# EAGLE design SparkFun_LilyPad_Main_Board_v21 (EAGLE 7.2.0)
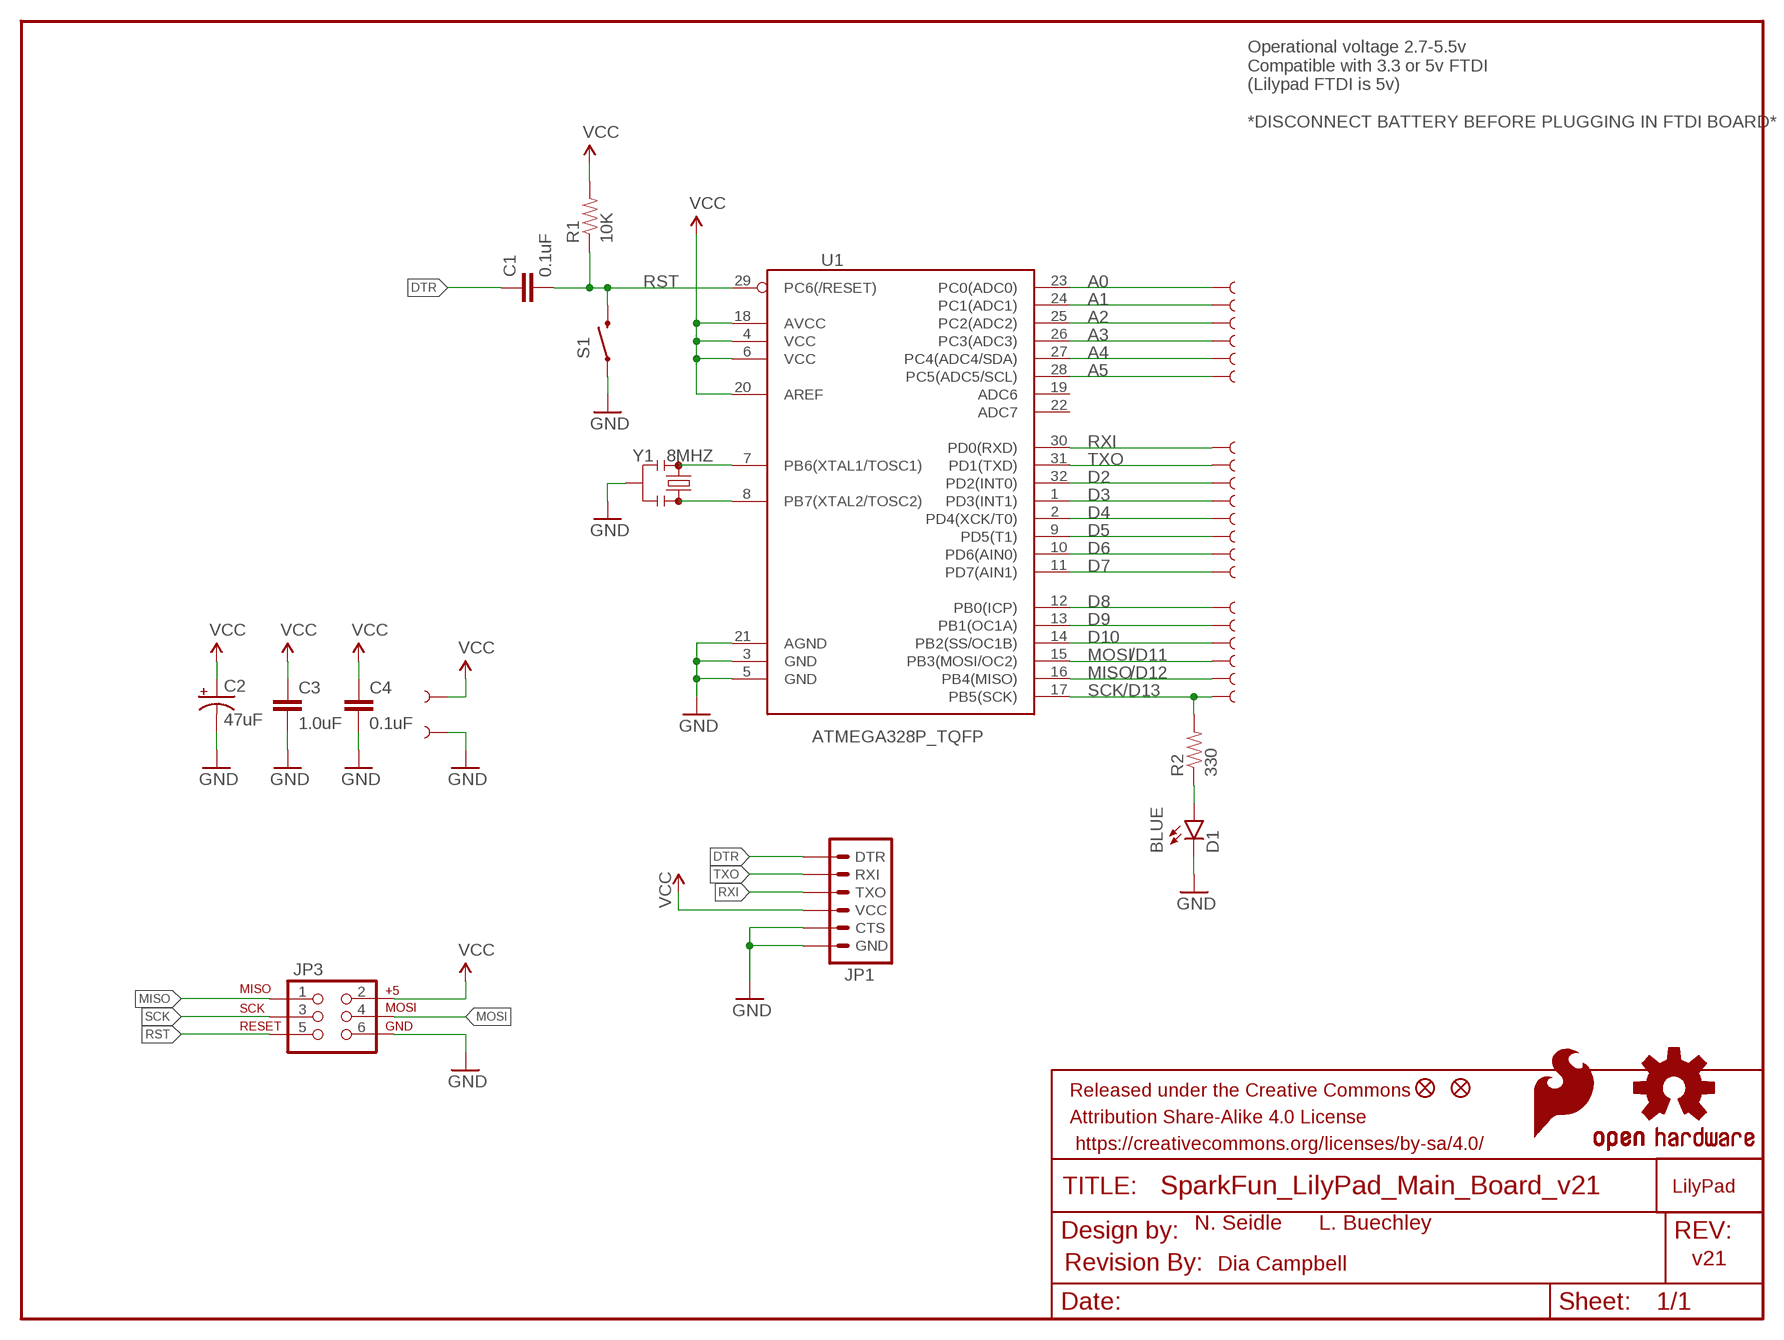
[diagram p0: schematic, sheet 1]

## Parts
$0000003  LOGO-LPLPA  [LOGO-LPA]
C1  0.1uF  0.1UF-25V(+80/-20%)(0603)  [0603-CAP]
C2  47uF  47UF-10V-10%(TANT)  [EIA3528]
C3  1.0uF  1.0UF-16V-10%(0603)  [0603-CAP]
C4  0.1uF  0.1UF-25V(+80/-20%)(0603)  [0603-CAP]
D1  BLUE  LED-BLUE0603  [LED-0603]
FID1  FIDUCIALUFIDUCIAL  [MICRO-FIDUCIAL]
FID2  FIDUCIALUFIDUCIAL  [MICRO-FIDUCIAL]
FRAME1  FRAME-LETTER  [CREATIVE_COMMONS]
GND  SEWTAP9  [PETAL-LONG-1-2SIDE]
JP1  ARDUINO_SERIAL_PROGRAMSMD  [1X06-SMD]
JP3  FEMALE 2x3  AVR_SPI_PRG_6NS  [2X3-NS]
LOGO1  SFE_LOGO_FLAME.3COP  [SFE_LOGO_FLAME_COPPER_.3]
LOGO2  OSHW-LOGO-COPPERM  [OSHW-LOGO-M]
R1  10K  10KOHM-1/10W-1%(0603)0603  [0603-RES]
R2  330  330OHM1/10W1%(0603)  [0603-RES]
S1  SWITCH-MOMENTARY-2SMD-REDUNDANT  [TACTILE-SWITCH-SMD]
U1  ATMEGA328P_TQFP  [TQFP32-08]
U$1  SEWTAP9  [PETAL-LONG-1-2SIDE]
U$2  SEWTAP9  [PETAL-LONG-1-2SIDE]
U$3  SEWTAP9  [PETAL-LONG-1-2SIDE]
U$4  SEWTAP9  [PETAL-LONG-1-2SIDE]
U$5  SEWTAP9  [PETAL-LONG-1-2SIDE]
U$6  SEWTAP9  [PETAL-LONG-1-2SIDE]
U$7  SEWTAP9  [PETAL-LONG-1-2SIDE]
U$8  SEWTAP9  [PETAL-LONG-1-2SIDE]
U$9  SEWTAP9  [PETAL-LONG-1-2SIDE]
U$10  SEWTAP9  [PETAL-LONG-1-2SIDE]
U$11  SEWTAP9  [PETAL-LONG-1-2SIDE]
U$12  SEWTAP9  [PETAL-LONG-1-2SIDE]
U$13  SEWTAP9  [PETAL-LONG-1-2SIDE]
U$14  SEWTAP9  [PETAL-LONG-1-2SIDE]
U$15  SEWTAP9  [PETAL-LONG-1-2SIDE]
U$16  SEWTAP9  [PETAL-LONG-1-2SIDE]
U$17  SEWTAP9  [PETAL-LONG-1-2SIDE]
U$18  SEWTAP9  [PETAL-LONG-1-2SIDE]
U$19  SEWTAP9  [PETAL-LONG-1-2SIDE]
U$20  SEWTAP9  [PETAL-LONG-1-2SIDE]
U$21  SEWTAP9  [PETAL-LONG-1-2SIDE]
U$22  REVISION  [REVISION]
Y1  8MHZ  RESONATOR8MHZ  [RESONATOR-SMD]

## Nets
A0: U1.23(PC0(ADC0)) U$1.1
A1: U1.24(PC1(ADC1)) U$2.1
A2: U1.25(PC2(ADC2)) U$3.1
A3: U1.26(PC3(ADC3)) U$4.1
A4: U1.27(PC4(ADC4/SDA)) U$5.1
A5: U1.28(PC5(ADC5/SCL)) U$6.1
D2: U1.32(PD2(INT0)) U$9.1
D3: U1.1(PD3(INT1)) U$10.1
D4: U1.2(PD4(XCK/T0)) U$11.1
D5: U1.9(PD5(T1)) U$12.1
D6: U1.10(PD6(AIN0)) U$13.1
D7: U1.11(PD7(AIN1)) U$14.1
D8: U1.12(PB0(ICP)) U$15.1
D9: U1.13(PB1(OC1A)) U$16.1
D10: U1.14(PB2(SS/OC1B)) U$17.1
DTR: C1.1 JP1.1(DTR)
GND [VCC]: C2.C(-) C3.2 C4.2 D1.C GND.1 JP1.5(CTS) JP1.6(GND) JP3.6 S1.1 S1.2 U1.3(GND) U1.5(GND) U1.21(AGND) Y1.2
MISO: JP3.1 U1.16(PB4(MISO)) U$19.1
MOSI: JP3.4 U1.15(PB3(MOSI/OC2)) U$18.1
N$1: U1.7(PB6(XTAL1/TOSC1)) Y1.1
N$2: D1.A R2.1
N$3: U1.8(PB7(XTAL2/TOSC2)) Y1.3
RST: C1.2 JP3.5 R1.1 S1.3 S1.4 U1.29(PC6(/RESET))
RXI: JP1.3(TXO) U1.30(PD0(RXD)) U$7.1
SCK: JP3.3 R2.2 U1.17(PB5(SCK)) U$21.1
TXO: JP1.2(RXI) U1.31(PD1(TXD)) U$8.1
VCC [VCC]: C2.A(+) C3.1 C4.1 JP1.4(VCC) JP3.2 R1.2 U1.4(VCC) U1.6(VCC) U1.18(AVCC) U1.20(AREF) U$20.1
Unconnected: U1.19(ADC6) U1.22(ADC7)

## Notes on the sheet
- Operational voltage 2.7-5.5v
  Compatible with 3.3 or 5v FTDI
  (Lilypad FTDI is 5v)
  
  *DISCONNECT BATTERY BEFORE PLUGGING IN FTDI BOARD*
- /D11
- /D12
- /D13
- N. Seidle | L. Buechley
- Dia Campbell | v21

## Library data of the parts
$0000003 = LilyPad-Wearables:LOGO-LP
C1 C4 = SparkFun-Capacitors:0.1UF-25V(+80/-20%)(0603): CAP-00810; PROD_ID: CAP-00810
C2 = SparkFun-Capacitors:47UF-10V-10%(TANT): CAP-08310; PROD_ID: CAP-08310
C3 = SparkFun-Capacitors:1.0UF-16V-10%(0603): CAP-00868; PROD_ID: CAP-00868
D1 = SparkFun-LED:LED-BLUE: Blue LEDs for production use; PROD_ID: DIO-08575
FID1 FID2 = SparkFun-Aesthetics:FIDUCIAL: Fiducial Alignment Points
FRAME1 = SparkFun-Aesthetics:FRAME-LETTER: Schematic Frame; DESIGNER: NAME; VERSION: v01
GND U$1-U$21 = LilyPad-Wearables:SEWTAP: Sew Taps for LilyPad Boards.
JP1 = SparkFun-Connectors:ARDUINO_SERIAL_PROGRAM: FTDI connector footprints; PROD_ID: CONN-08971
JP3 = SparkFun-Connectors:AVR_SPI_PRG_6: AVR ISP 6 Pin This is the reduced ISP connector for AVR programming. Common on Arduino. This footprint will take up less PCB space and can be used with a 10-pin to 6-pin adapter such as SKU: BOB-08508 **Special note about "TEST_POINT" package. The stop mask is on the top side, so if you want your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
LOGO1 = SparkFun-Aesthetics:SFE_LOGO_FLAME: SFE Logo, flame only
LOGO2 = SparkFun-Aesthetics:OSHW-LOGO-COPPER: Open Source Hardware Logo
R1 = SparkFun-Resistors:10KOHM-1/10W-1%(0603): RES-00824; PROD_ID: RES-00824
R2 = SparkFun-Resistors:330OHM1/10W1%(0603): RES-00818; PROD_ID: RES-00818
S1 = SparkFun-Electromechanical:SWITCH-MOMENTARY-2: Various NO switches- pushbuttons, reed, etc; PROD_ID: SWCH-08247
U1 = SparkFun-DigitalIC:ATMEGA328P_TQFP; PROD_ID: IC-09069
U$22 = SparkFun-Aesthetics:REVISION
Y1 = SparkFun-FreqCtrl:RESONATOR: Resonator Small SMD resonator. Used, eg, on the Arduino Pro/ Pro Mini boards. 8MHz- XTAL-08895 16MHz- XTAL-08900; PROD_ID: XTAL-08895

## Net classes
0 Default: width 0.203 mm
1 VCC: width 0.305 mm

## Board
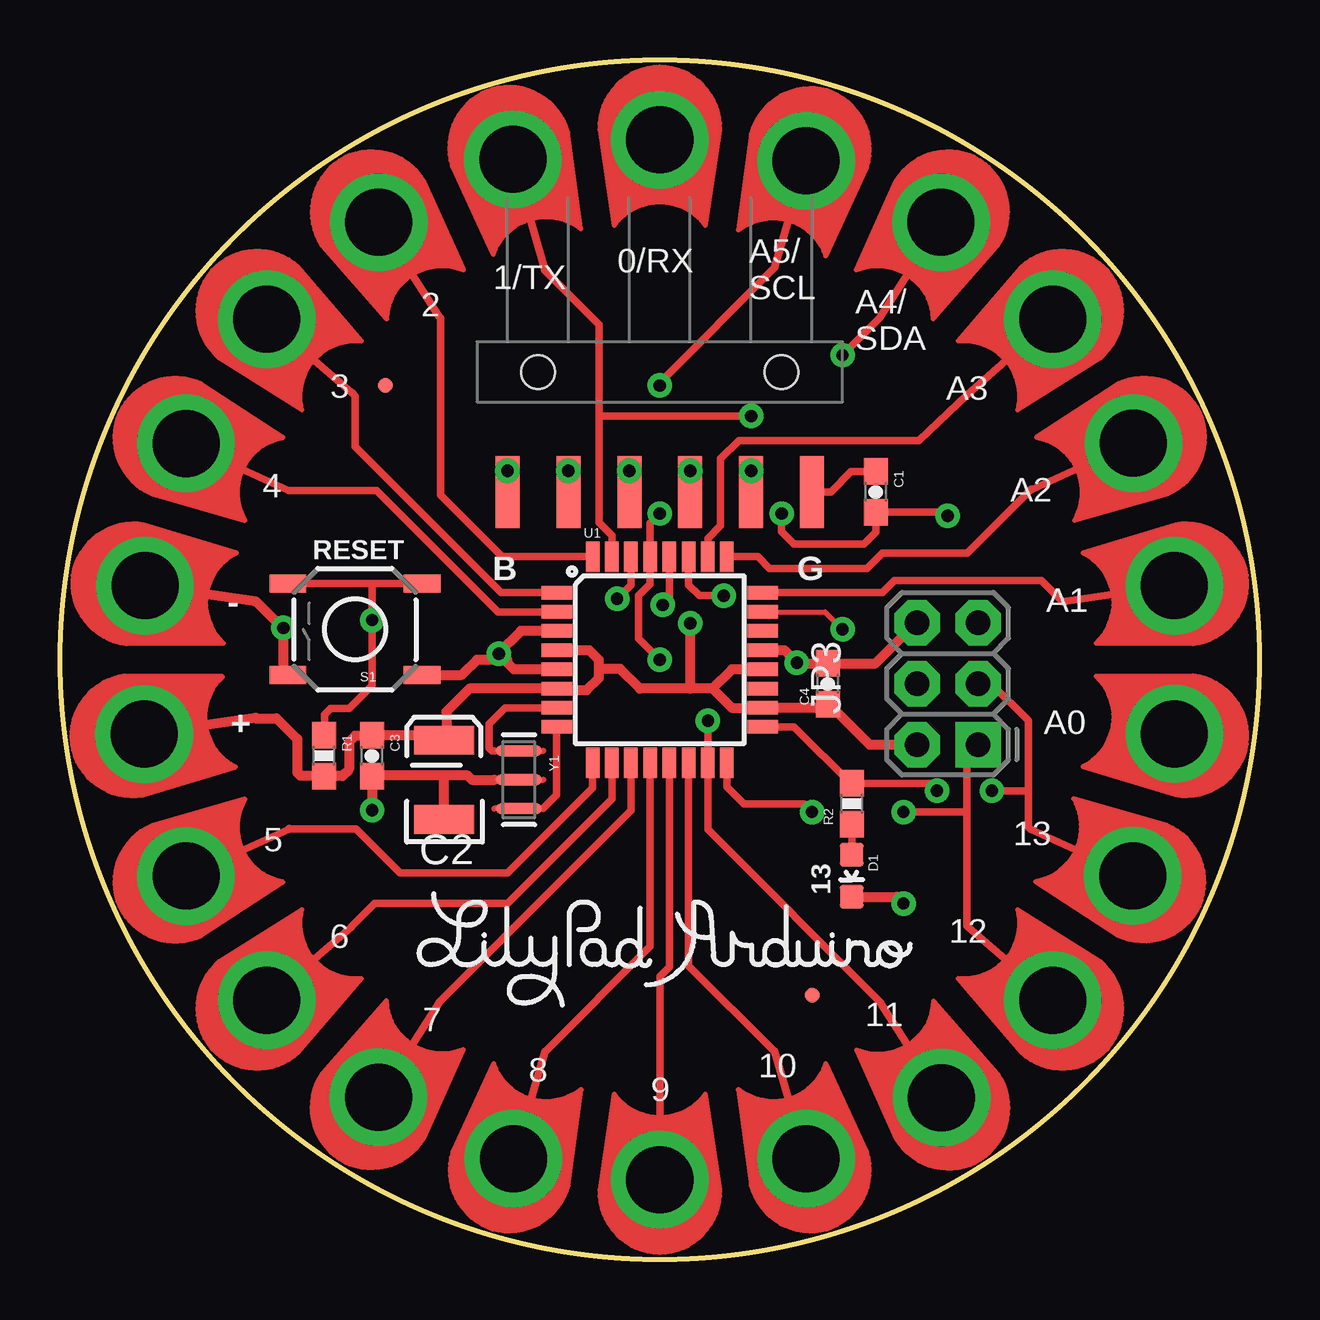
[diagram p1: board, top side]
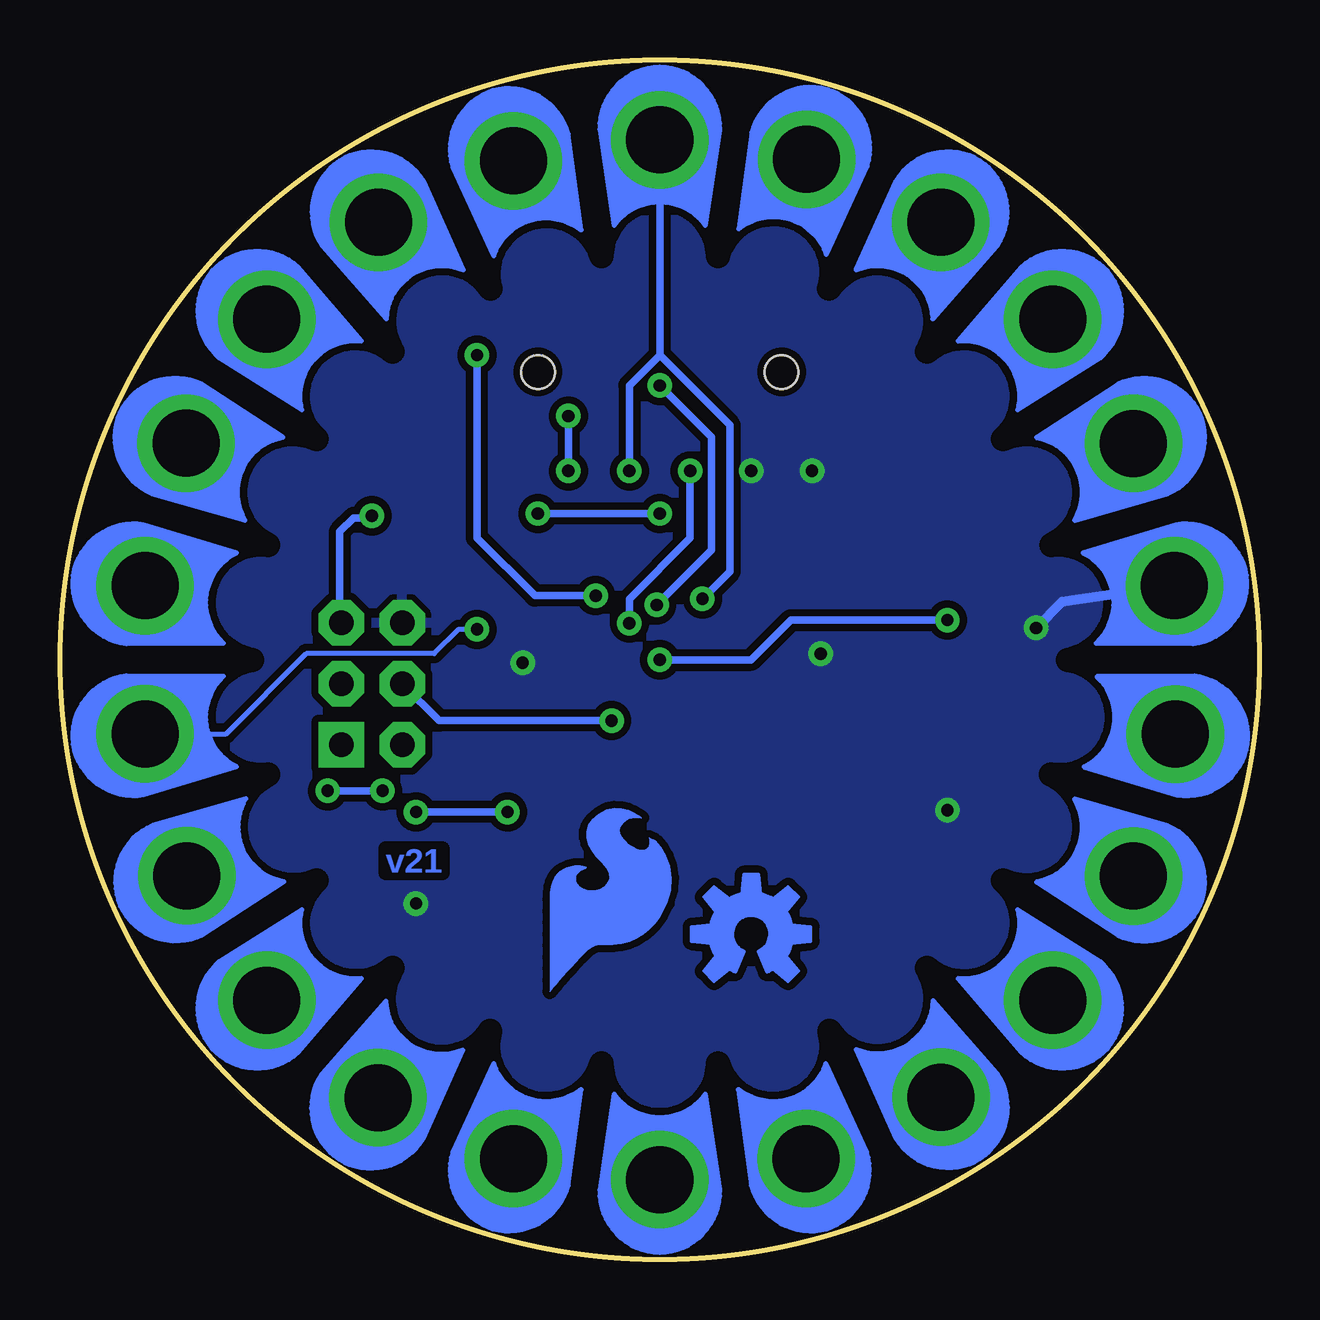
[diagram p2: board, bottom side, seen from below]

Size 50 x 50 mm. Coordinates in mm from the lower left corner, seen from the top.
Outline: circle at 25,25 radius 25
Copper layers (1*16): Top 0.035mm / dielectric 1.5mm / Bottom 0.035mm
Design rules "SparkFun-2-layer": minimum track width 7mil, minimum drill 15mil, track to track 8mil, track to pad 8mil, pad to pad 8mil, via to via 8mil, smd to smd 8mil, copper to edge 8mil, drill to drill 8mil, minimum pad ring 12mil, minimum via ring 10mil, stop-mask expansion 4mil, vias tented up to drill 20mil, thermal gap 10mil
bRestrict: area 2.4,2.4 to 47.6,47.6; area 21,42.8 to 23.5,44; area 31.6,41.3 to 34.4,43; area 36.3,38.4 to 38.9,40.7; area 40,34.1 to 42,36.9; area 42.2,29.2 to 43.6,31.8; area 42.8,23.9 to 44,26.2; area 42.2,18.2 to 43.7,20.9; area 36.3,9.4 to 39,11.7; area 31.7,7 to 34.5,8.7; area 26.5,6 to 28.9,7.3; area 21.1,6 to 23.6,7.3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; 22 lines

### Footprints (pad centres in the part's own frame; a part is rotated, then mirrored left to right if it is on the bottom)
0603-CAP = smd 1.1 x 1: 1 -0.85,0; 2 0.85,0
EIA3528 = smd 1.2 x 2.5: A 1.65,0; C -1.65,0
LED-0603 = smd 1 x 1: A 0,-0.877; C 0,0.877
MICRO-FIDUCIAL = smd 0.635 x 0.635: 1 0,0
PETAL-LONG-1-2SIDE = drill 2.794 pad 4.064: 1 0.03,0
1X06-SMD = smd 1 x 3: 1 -6.35,5; 2 -3.81,5; 3 -1.27,5; 4 1.27,5; 5 3.81,5; 6 6.35,5 | hole 1.4: -5.08,0; 5.08,0
2X3-NS = drill 1.016 pad 1.88 square: 1 -2.54,-1.27 | drill 1.016 pad 1.88 octagon: 2 -2.54,1.27; 3 0,-1.27; 4 0,1.27; 5 2.54,-1.27; 6 2.54,1.27
0603-RES = smd 1.1 x 1: 1 -0.85,0; 2 0.85,0
TACTILE-SWITCH-SMD = smd 1.524 x 0.762: 1 -2.794,1.905; 2 2.794,1.905; 3 -2.794,-1.905; 4 2.794,-1.905
TQFP32-08 = smd 1.27 x 0.559: 1 -4.293,2.8; 2 -4.293,2; 3 -4.293,1.2; 4 -4.293,0.4; 5 -4.293,-0.4; 6 -4.293,-1.2; 7 -4.293,-2; 8 -4.293,-2.8; 17 4.293,-2.8; 18 4.293,-2; 19 4.293,-1.2; 20 4.293,-0.4; 21 4.293,0.4; 22 4.293,1.2; 23 4.293,2; 24 4.293,2.8 | smd 0.559 x 1.27: 9 -2.8,-4.293; 10 -2,-4.293; 11 -1.2,-4.293; 12 -0.4,-4.293; 13 0.4,-4.293; 14 1.2,-4.293; 15 2,-4.293; 16 2.8,-4.293; 25 2.8,4.293; 26 2,4.293; 27 1.2,4.293; 28 0.4,4.293; 29 -0.4,4.293; 30 -1.2,4.293; 31 -2,4.293; 32 -2.8,4.293
RESONATOR-SMD = smd 0.45 x 1.905: 1 -1.2,0; 2 0,0; 3 1.2,0

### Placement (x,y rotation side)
$0000003  25,13.3 0 top
C1  34,32 270 top
C2  16,20 90 top
C3  13,21 270 top
C4  32,24 90 top
D1  33,16 180 top
FID1  13.57,36.43 0 top
FID2  31.35,11.03 0 top
FRAME1  not placed on the board
GND  3.52,28.09 351.8 top
JP1  25,37 180 top
JP3  37,24 90 top
LOGO1  30.08,11.03 0 bottom
LOGO2  21.19,13.57 0 bottom
R1  11,21 270 top
R2  33,19 90 top
S1  12.3,26.27 180 top
U1  25,25 0 top
U$1  46.48,21.91 171.8 top
U$2  46.48,28.09 188.2 top
U$3  44.77,34.04 204.5 top
U$4  41.4,39.21 220.9 top
U$5  36.74,43.26 237.3 top
U$6  31.11,45.83 253.7 top
U$7  25,46.7 270 top
U$8  18.87,45.89 286.3 top
U$9  13.27,43.26 302.7 top
U$10  8.6,39.21 319.1 top
U$11  5.23,34.03 335.5 top
U$12  5.23,15.97 24.5 top
U$13  8.6,10.79 40.9 top
U$14  13.26,6.74 57.3 top
U$15  18.89,4.17 73.7 top
U$16  25,3.3 90 top
U$17  31.11,4.17 106.3 top
U$18  36.76,6.72 122.7 top
U$19  41.4,10.79 139.1 top
U$20  3.48,21.9 8.2 top
U$21  44.74,15.98 155.5 top
U$22  not placed on the board
Y1  19.13,20 270 top

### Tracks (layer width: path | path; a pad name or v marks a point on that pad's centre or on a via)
A0  (via drill 0.51)
  Top 0.203: U1.23 31.89,27 v32.62,26.27
  Bottom 0.203: v32.62,26.27 33.38,26.27 34.4,25.25 39.73,25.25 43.07,21.91 U$1.1
A1
  Top 0.305: U$2.1 41.83,27.42 41.82,27.42 41.8,27.4 40.9,28.3 34.78,28.3 34.28,27.8 U1.24
A2
  Top 0.305: U$3.1 40.5,32.1 40.5,32.11 40.49,32.11 37.83,29.45 34.27,29.45 33.64,28.81 29.57,28.81 29.09,29.29 U1.25
A3
  Top 0.305: U1.26 27,30.05 27.54,30.59 27.54,33.38 28.3,34.14 35.8,34.14 37.83,36.05 U$4.1
A4  (via drill 0.51)
  Top 0.305: U$5.1 34.2,39.3 34.2,39.28 v32.62,37.7 | U1.27 26.2,28.12 26.65,27.67 v27.67,27.67
  Bottom 0.305: v27.67,27.67 30.21,27.67 32.62,30.08 v32.62,37.7
A5  (via drill 0.51)
  Top 0.305: U$6.1 29.8,41.4 29.8,41.36 25,36.56 v25,36.43 | U1.28 25.4,27.56 v25.13,27.29
  Bottom 0.305: v25,36.43 22.84,34.27 22.84,29.57 v25.13,27.29
D2
  Top 0.305: U$9.1 15.8,39.3 15.86,39.24 15.86,31.86 18.42,29.29 U1.32
D3
  Top 0.305: U$10.1 12.16,36.13 12.17,36.13 12.3,36 12.3,33.89 18.39,27.8 U1.1
D4
  Top 0.305: U$11.1 9.54,32.06 9.56,32.06 13.19,32.06 18.25,27 U1.2
D5
  Top 0.305: U$12.1 9.54,17.93 9.54,17.95 9.56,17.96 9.58,17.94 12.35,17.94 14.18,16.11 18.65,16.11 22.2,19.66 U1.9
D6
  Top 0.305: U$13.1 12.15,13.87 12.15,13.88 13.11,14.84 18.65,14.84 23,19.19 U1.10
D7
  Top 0.305: U$14.1 15.8,10.7 15.8,10.72 23.8,18.72 U1.11
D8
  Top 0.305: U$15.1 20.21,8.68 20.24,8.68 24.6,13.04 U1.12
D9
  Top 0.305: 25,11.79 U$16.1 | 25,11.79 25,8 | U1.13 25.4,12.19 25,11.79
D10
  Top 0.305: U$17.1 29.79,8.69 29.75,8.69 26.2,12.24 U1.14
DTR
  Top 0.305: JP1.1 32.13,32 32.98,32.85 C1.1
GND  (via drill 0.51)
  Top 0.305: C4.2 32,24.8 | v13,18.74 v13.01,18.73 | C2.C 16,18.41 16.03,18.45 15.98,18.5 | v18.29,25.25 18.32,25.28 | 13.06,20.17 13.04,20.15 C3.2 | 18.27,25.25 v18.29,25.25 | JP1.6 v18.65,32.87 | JP1.5 v21.19,32.87 | 9.3,26.3 9.31,26.31 v9.31,26.33 9.27,26.33 | 8.18,27.42 8.17,27.42 | 9.3,24.57 S1.2 | v18.29,25.25 18.4,25.25 18.65,25
  Top 0.406: 8.17,27.42 GND.1 | C3.2 v13,18.74 | 15.98,20.17 17,20.17 17.17,20 18.11,20 | 15.98,20.17 15.98,18.5 | 15.98,20.17 13.06,20.17 | 9.27,26.33 8.18,27.42 | U1.5 18.92,24.6 18.27,25.25 19.21,26.2 U1.3 | U1.21 30.19,25.4 v30.71,24.87 30.74,24.85 C4.2 33.99,24.85 35.67,26.52 | 9.3,26.3 9.3,24.57 | 18.65,25 17.38,25 16.74,24.36 S1.1 | D1.C 34.88,15.12 v35.16,14.84
  Bottom 0.406: GND.1 8.24,27.41 v9.31,26.33
  pour Bottom (isolate 0.305): -1,51 51,51 51,-1 -1,-1
MISO  (via drill 0.51)
  Top 0.305: U$19.1 37.85,13.87 37.82,13.9 37.8,13.9 37.8,18.65 | JP3.1 37.8,20.99 37.8,18.65 | U1.16 27.8,19.7 28.5,19 31,19 v31.35,18.65 | v35.16,18.65 37.8,18.65
  Bottom 0.305: v31.35,18.65 v35.16,18.65
MOSI  (via drill 0.51)
  Top 0.305: U$18.1 34.2,10.7 34.2,10.72 27,17.92 U1.15 v27,22.45 v27.01,22.46
  Bottom 0.305: JP3.4 35.74,24.01 | JP3.4 | v27.01,22.46 34.2,22.46 JP3.4
N$1
  Top 0.305: U1.7 18.55,23 17.89,22.33 17.89,21.32 18,21.2 18.11,21.2
N$2
  Top 0.305: 33,16.7 D1.A R2.1
N$3
  Top 0.305: U1.8 20.71,19.36 20.14,18.8
RST  (via drill 0.51)
  Top 0.305: R1.1 11.03,21.82 11.03,22.71 11.28,22.97 12.05,22.97 13.01,23.93 v13.01,26.65 13.01,28.1 12.94,28.18 | v37,31 36.85,31.15 C1.2 34,30.32 33.51,29.83 30.59,29.83 30.08,30.33 v30.08,31.1 | v25,25 24.11,25.89 24.11,27.67 24.6,28.16 U1.29 24.6,30.7 v25,31.1 | S1.4 12.94,28.18 | 12.94,28.18 S1.3
  Bottom 0.305: v25,25 21.19,25 19.54,26.65 v13.01,26.65 12.94,26.65 | v37,31 37,30.91 37.76,30.91 38.34,30.33 38.34,26.61 JP3.5 | v25,31.1 v30.08,31.1
RXI  (via drill 0.51)
  Top 0.254: 26.27,31.98 JP1.3 v26.27,32.87
  Top 0.305: U1.30 23.8,28.12 v23.22,27.54
  Bottom 0.305: 25,37.7 U$7.1 | v26.27,32.87 26.27,36.43 25,37.7 | v23.22,27.54 22.08,28.68 22.08,34.78 25,37.7
SCK  (via drill 0.51)
  Top 0.305: U$21.1 40.46,17.93 40.37,18.02 40.37,19.6 | U1.17 30.6,22.2 33,19.8 R2.2 36.25,19.85 v36.56,19.54 | JP3.3 38.83,24 40.37,22.46 40.37,19.6 | v38.84,19.54 40.3,19.54 40.37,19.6
  Bottom 0.305: v36.56,19.54 v38.84,19.54
TXO  (via drill 0.51)
  Top 0.254: 28.81,31.98 JP1.2 v28.81,32.87
  Top 0.305: U1.31 23,30.18 22.46,30.71 22.46,35.16 | 22.46,35.16 22.46,38.97 20.2,41.23 20.2,41.3 U$8.1 | 22.46,35.16 v28.81,35.16
  Bottom 0.305: v28.81,35.16 v28.81,32.87
VCC  (via drill 0.51)
  Top 0.305: 8.16,22.56 8.17,22.57 8.17,22.58 | 10.57,20.15 R1.2 10.98,20.17 | 15.7,21.85 15.91,21.65 C2.A 15.95,21.65 15.9,21.7 | C4.1 32,23.1 31.9,23 | C4.1 32.05,23.15 | 12.94,21.82 12.96,21.85 C3.1 | v23.73,32.87 JP1.4 | 31.85,23 C4.1 | 21.19,23.73 21.12,23.8 U1.6 | 22.59,24.62 22.46,24.49
  Top 0.406: 8.17,22.58 U$20.1 | 15.7,21.85 C3.1 | 27.2,23.8 28,24.6 U1.20 | 27.2,23.8 28,23 U1.18 31.85,23 | JP3.2 33.74,21.46 32.05,23.15 | R1.2 11.77,20.15 12.05,20.43 12.05,21.57 12.3,21.82 12.94,21.82 | 21.19,23.73 21.95,23.73 22.46,24.24 22.46,24.49 22.46,25 22.06,25.4 U1.4 | v26.27,26.52 26.27,23.8 | 27.2,23.8 26.27,23.8 | 26.27,23.8 24.17,23.8 23.35,24.62 22.59,24.62 | 8.16,22.56 9.02,22.56 9.89,21.7 9.89,20.3 10.01,20.17 10.98,20.17 | U1.6 17.07,23.8 16.11,22.84 16.11,21.76 C2.A
  Bottom 0.305: v26.27,26.52 26.27,27.54 23.73,30.08 v23.73,32.87

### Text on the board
Bottom: v21
tPlace: 0/RX | 1/TX | A5/ / SCL | 2 | A4/ / SDA | 3 | A3 | 4 | A2 | RESET | B | G | - | A1 | + | A0 | 5 | 13 | 13 | 6 | 12 | 11 | 7 | 10 | 8 | 9
Measures: dimensions in inches
tDocu: purple 0.8 mm | L. Buechley | N. Seidle | Dia Campbell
